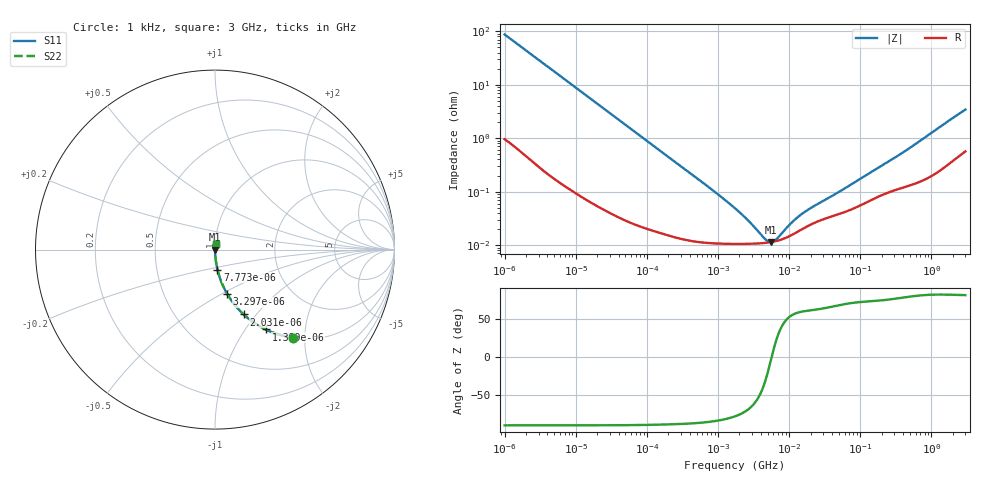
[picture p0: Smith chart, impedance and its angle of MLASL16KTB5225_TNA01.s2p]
! MLASL16KTB5225_TNA01  S-PARAMETER MODEL  ( Standard Model )
! Model Generated by TAIYO YUDEN Corporation (http://www.ty-top.com)
! Version 1.0
! TAIYO YUDEN Control No. 220601
! Copyright(c) 2009 TAIYO YUDEN CO.,LTD. All Rights Reserved.
! Product Description (link to TY-COMPAS)
! https://ds.yuden.co.jp/TYCOMPAS/or/detail?pn=MLASL16KTB5225KTNA01&u=M
! Products Name : Multilayer Ceramic Capacitors
! Characteristics :
!  Capacitance : 2.2 [uF] , Rated Voltage : 10 [V] , TCC : X5R
!  Case Size : 1.6 x 0.8 / 0.063 x 0.031 [mm/inch] , Thickness : 0.45 / 0.018 [mm/inch]
!  (Conditions: Temperature = 25 [degC] , DC Bias Voltage = 0 [V])
! External Node Assignments :
!  1  o---| |---o  2
! GND o---------o GND
! Frequency Range : 1kHz  -  3GHz  [ 401 STEP ]
# MHZ S RI R 50
! Freq[MHz].  S11 Real  S11 Imag  S21 Real  S21 Imag  S12 Real  S12 Imag  S22 Real  S22 Imag
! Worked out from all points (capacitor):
!   401 points, 1 kHz to 3 GHz, reference 50 ohm
!   read as one part in series: C = 1.82 uF near 1.077 kHz
!   lowest |Z| = 11.4 mohm at 5.502 MHz (marker M1)
!   series resonance near 5.681 MHz, so ESL is about 430 pH
!   S11 on the Smith chart (normalised r, x): 1 kHz: 1.02, -1.74; 1.399 kHz: 1.01, -1.25; 2.031 kHz: 1.01, -0.86; 3.297 kHz: 1.01, -0.53; 7.773 kHz: 1.00, -0.23; 3 GHz: 1.01, +0.07
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0.001  0.4326 -0.49  0.5674 0.49  0.5674 0.49  0.4326 -0.49
0.001399  0.2832 -0.4451  0.7168 0.4451  0.7168 0.4451  0.2832 -0.4451
0.002031  0.1598 -0.3612  0.8402 0.3612  0.8402 0.3612  0.1598 -0.3612
0.003297  0.0685 -0.2478  0.9315 0.2478  0.9315 0.2478  0.0685 -0.2478
0.007773  0.0139 -0.112  0.9861 0.112  0.9861 0.112  0.0139 -0.112
0.01216  0.00606 -0.0723  0.9939 0.0723  0.9939 0.0723  0.00606 -0.0723
0.033275  0.00109 -0.0267  0.9989 0.0267  0.9989 0.0267  0.00109 -0.0267
0.147855  0.000208 -0.00609  0.9998 0.00609  0.9998 0.00609  0.000208 -0.00609
0.734727  0.000111 -0.00122  0.9999 0.00122  0.9999 0.00122  0.000111 -0.00122
1.732051  0.000106 -0.000478  0.9999 0.000478  0.9999 0.000478  0.000106 -0.000478
2.709407  0.000106 -0.00026  0.9999 0.00026  0.9999 0.00026  0.000106 -0.00026
4.566395  0.00011 -7.09e-05  0.9999 7.09e-05  0.9999 7.09e-05  0.00011 -7.09e-05
5.106836  0.000112 -3.44e-05  0.9999 3.44e-05  0.9999 3.44e-05  0.000112 -3.44e-05
5.502215  0.000114 -1.03e-05  0.9999 1.03e-05  0.9999 1.03e-05  0.000114 -1.03e-05
5.928204  0.000116 1.38e-05  0.9999 -1.38e-05  0.9999 -1.38e-05  0.000116 1.38e-05
6.629817  0.00012 4.99e-05  0.9999 -4.99e-05  0.9999 -4.99e-05  0.00012 4.99e-05
9.991309  0.000146 0.000186  0.9999 -0.000186  0.9999 -0.000186  0.000146 0.000186
12.97096  0.000176 0.000276  0.9998 -0.000276  0.9998 -0.000276  0.000176 0.000276
21.06097  0.00025 0.000449  0.9998 -0.000449  0.9998 -0.000449  0.00025 0.000449
51.53541  0.000386 0.000935  0.9996 -0.000935  0.9996 -0.000935  0.000386 0.000935
256.0921  0.000992 0.0036  0.999 -0.0036  0.999 -0.0036  0.000992 0.0036
3000  0.00675 0.0334  0.9933 -0.0334  0.9933 -0.0334  0.00675 0.0334
